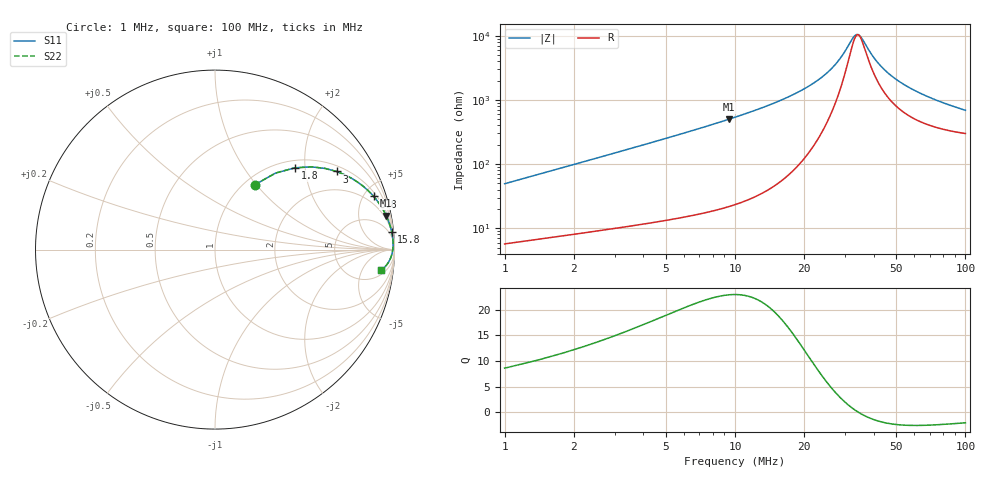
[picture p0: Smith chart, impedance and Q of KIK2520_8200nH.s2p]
!version-2
!date-01.2022
!Series
# MHz S RI R 50
!Freq ReS11 ImS11 ReS21 ImS21 ReS12 ImS12 ReS22 ImS22
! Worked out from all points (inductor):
!   249 points, 1 MHz to 100 MHz, reference 50 ohm
!   read as one part in series: L = 7.8 uH near 1.4 MHz
!   highest Q = 22.9 at 9.4 MHz (marker M1), where L = 8.44 uH
!   self-resonance near 34.2 MHz
!   S11 on the Smith chart (normalised r, x): 1 MHz: 1.11, +0.98; 1.8 MHz: 1.15, +1.77; 3 MHz: 1.20, +2.96; 5.8 MHz: 1.29, +5.86; 15.8 MHz: 2, +20; 100 MHz: 7, -12
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1  0.2216 0.3612  0.7784 -0.3612  0.7784 -0.3612  0.2216 0.3612
1.4  0.3377 0.4265  0.6623 -0.4265  0.6623 -0.4265  0.3377 0.4265
1.8  0.4455 0.4557  0.5545 -0.4557  0.5545 -0.4557  0.4455 0.4557
3  0.6771 0.4353  0.3229 -0.4353  0.3229 -0.4353  0.6771 0.4353
4.2  0.8009 0.3718  0.1991 -0.3718  0.1991 -0.3718  0.8009 0.3718
5.8  0.8841 0.2962  0.1159 -0.2962  0.1159 -0.2962  0.8841 0.2962
9.4  0.9538 0.1892  0.0462 -0.1892  0.0462 -0.1892  0.9538 0.1892
15.8  0.9845 0.0991  0.0155 -0.0991  0.0155 -0.0991  0.9845 0.0991
17.8  0.9879 0.0817  0.0121 -0.0817  0.0121 -0.0817  0.9879 0.0817
25.4  0.9923 0.0353  0.00772 -0.0353  0.00772 -0.0353  0.9923 0.0353
28.6  0.9922 0.021  0.00784 -0.021  0.00784 -0.021  0.9922 0.021
32.6  0.9911 0.00576  0.00888 -0.00576  0.00888 -0.00576  0.9911 0.00576
34.2  0.9905 0.000257  0.0095 -0.000257  0.0095 -0.000257  0.9905 0.000257
35.4  0.99 -0.00368  0.01 0.00368  0.01 0.00368  0.99 -0.00368
39.4  0.9878 -0.0158  0.0122 0.0158  0.0122 0.0158  0.9878 -0.0158
41.8  0.9863 -0.0225  0.0137 0.0225  0.0137 0.0225  0.9863 -0.0225
45.8  0.9835 -0.0327  0.0165 0.0327  0.0165 0.0327  0.9835 -0.0327
50.6  0.9797 -0.0438  0.0203 0.0438  0.0203 0.0438  0.9797 -0.0438
57.8  0.9733 -0.0585  0.0267 0.0585  0.0267 0.0585  0.9733 -0.0585
67  0.9641 -0.0745  0.0359 0.0745  0.0359 0.0745  0.9641 -0.0745
83.8  0.9456 -0.0976  0.0544 0.0976  0.0544 0.0976  0.9456 -0.0976
100  0.9267 -0.1139  0.0733 0.1139  0.0733 0.1139  0.9267 -0.1139
